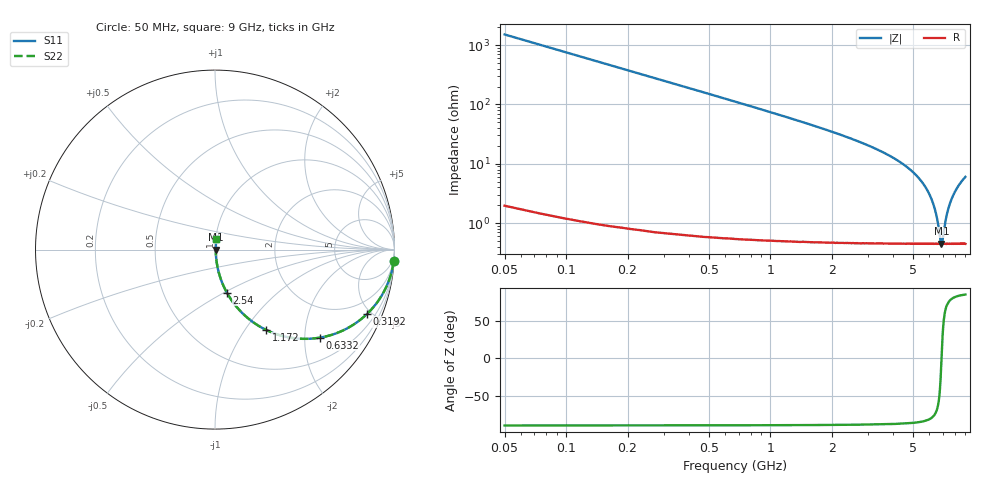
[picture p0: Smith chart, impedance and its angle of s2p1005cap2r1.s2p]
!	AVX	Thin	Film	Operation
!	Date:	March 2012
!	Description: Ultra-Miniature 01005 Size ACCU - P® Thin Film RF / Microwave Capacitor
!	Part Number:  C005YK2R1ABSTR
!	Serial	Measurements
#	MHz	S	db	R	50
!	S11	S21	S12	S22
!	dB	Phase	dB	Phase	dB	Phase	dB	Phase
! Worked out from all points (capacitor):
!   400 points, 50 MHz to 9 GHz, reference 50 ohm
!   read as one part in series: C = 2.1 pF near 94.86 MHz
!   lowest |Z| = 449 mohm at 6.869 GHz (marker M1)
!   series resonance near 6.878 GHz, so ESL is about 250 pH
!   S11 on the Smith chart (normalised r, x): 50 MHz: 1, -30; 319.2 MHz: 1.01, -4.74; 633.2 MHz: 1.01, -2.37; 1.172 GHz: 1.01, -1.26; 2.54 GHz: 1.01, -0.52; 9 GHz: 1.01, +0.12
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50  -0.02 -3.8  -23.63 86.2  -23.63 86.2  -0.02 -3.8
94.862  -0.07 -7.1  -18.12 82.8  -18.12 82.8  -0.07 -7.1
139.724  -0.15 -10.4  -14.83 79.5  -14.83 79.5  -0.15 -10.4
207.018  -0.32 -15.3  -11.58 74.6  -11.58 74.6  -0.32 -15.3
319.173  -0.72 -22.9  -8.21 67.0  -8.21 67.0  -0.72 -22.9
453.759  -1.35 -31.0  -5.77 58.8  -5.77 58.8  -1.35 -31.0
633.208  -2.35 -40.0  -3.84 49.7  -3.84 49.7  -2.35 -40.0
879.95  -3.82 -49.5  -2.38 40.1  -2.38 40.1  -3.82 -49.5
1171.554  -5.51 -57.5  -1.48 32.0  -1.48 32.0  -5.51 -57.5
1552.882  -7.56 -64.7  -0.88 24.7  -0.88 24.7  -7.56 -64.7
2539.85  -12.09 -74.6  -0.32 14.4  -0.32 14.4  -12.09 -74.6
3055.764  -14.22 -77.5  -0.21 11.2  -0.21 11.2  -14.22 -77.5
4536.216  -20.57 -81.9  -0.08 5.4  -0.08 5.4  -20.57 -81.9
5411.028  -25.48 -82.2  -0.05 3.0  -0.05 3.0  -25.48 -82.2
6016.667  -30.53 -79.7  -0.04 1.7  -0.04 1.7  -30.53 -79.7
6465.288  -36.90 -71.1  -0.04 0.8  -0.04 0.8  -36.90 -71.1
6869.048  -47.02 -3.5  -0.04 0.0  -0.04 0.0  -47.02 -3.5
6936.341  -46.33 22.6  -0.04 -0.1  -0.04 -0.1  -46.33 22.6
7250.376  -38.12 68.3  -0.04 -0.7  -0.04 -0.7  -38.12 68.3
7519.549  -33.94 76.1  -0.04 -1.1  -0.04 -1.1  -33.94 76.1
8125.188  -28.64 81.0  -0.04 -2.1  -0.04 -2.1  -28.64 81.0
9000  -24.47 82.3  -0.05 -3.4  -0.05 -3.4  -24.47 82.3
